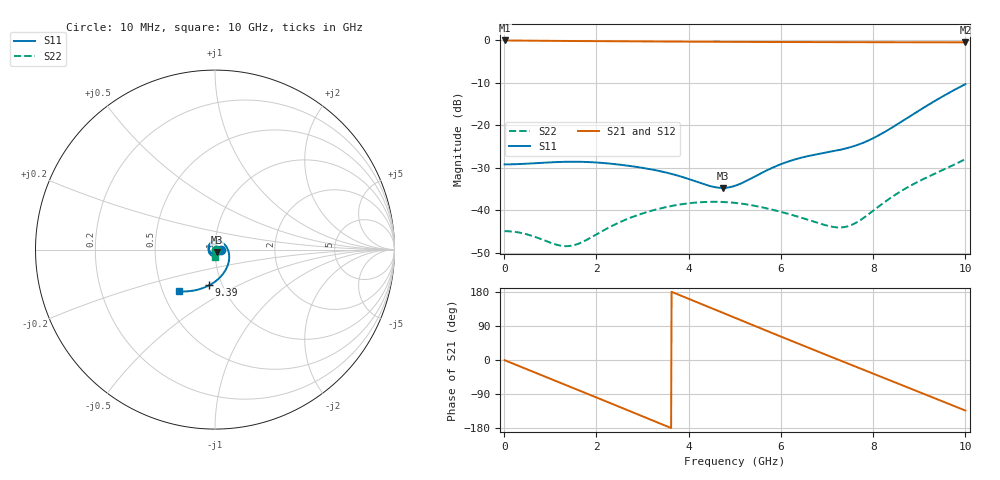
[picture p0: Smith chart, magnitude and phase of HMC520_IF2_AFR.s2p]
! Analog Devices, Inc.
! 1 Analog Way
! Wilmington, MA 01887
! http://www.analog.com
! Date:  2021-09-07 NN
! Board Name:  EV1HMC520ALC4 Revision A with HMC520ALC4 installed
! File Description:  Automatic Fixture Removal S-Parameters for IF2 Port connector and board loss de-embedding
! File Generation:  Calibrated Network Analyzer
! Chip Part Number:  HMC520A
! Chip Description:  GaAs, MMIC, IQ Mixer
! Chip Frequency:  6 to 10 GHz
! Chip Package:  LCC, 3.9 x 3.9 x 0.9 mm
! IF2 Port:  HMC520ALC4 removed and end of trace left open
!Note:
!  Analog Devices supplies this data as a sample of measured data at the evaluation board
!  ports for this product.  Your particular data for this product may vary.
!  Analog Devices reserves the right to change this data at anytime.
!  All lines below in this file are as is from the Network Analyzer.
!Agilent Technologies,N5245A,MY52451809,A.10.47.06
!Automatic Fixture Removal (AFR)
!Date: Friday, August 27, 2021 5:03:51 AM
!S2P File: Measurements: S11,S21,S12,S22:
# MHz S  RI  R 50
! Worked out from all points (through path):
!   1000 points, 10 MHz to 10 GHz, reference 50 ohm
!   highest |S21| = 0.00 dB at 10 MHz (marker M1); lowest = -0.4 dB at 10 GHz (marker M2)
!   group delay of S21, straight-line fit = 137 ps
!   lowest |S11| = -34.7 dB at 4.74 GHz (marker M3), VSWR 1.04, Z = 51.3 - j1.32 ohm
!   |S11| at or under -10 dB: start of sweep to end of sweep
!   |S22| runs from -48.4 to -27.9 dB; largest |S21 - S12| = 1.4e-15
!   S11 on the Smith chart (normalised r, x): 10 MHz: 1.07, -0.00; 9.39 GHz: 0.87, -0.36; 10 GHz: 0.61, -0.31
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10  0.0348 -0.000509  0.9999 -0.0086  0.9999 -0.0086  0.00571 -8.85e-05
750  0.0172 -0.0318  0.7924 -0.5968  0.7924 -0.5968  0.00153 -0.00446
1230  -0.00554 -0.0368  0.4833 -0.8607  0.4833 -0.8607  -0.00252 -0.00292
1680  -0.025 -0.0277  0.1209 -0.9767  0.1209 -0.9767  -0.00409 0.00101
2060  -0.0344 -0.0123  -0.2004 -0.9609  -0.2004 -0.9609  -0.00302 0.00454
2440  -0.0345 0.00557  -0.4991 -0.8421  -0.4991 -0.8421  -0.000141 0.007
2910  -0.0225 0.0232  -0.7897 -0.5724  -0.7897 -0.5724  0.00465 0.00757
3340  -0.00473 0.0289  -0.9413 -0.2429  -0.9413 -0.2429  0.00888 0.00544
4010  0.0178 0.0151  -0.9146 0.3159  -0.9146 0.3159  0.012 -0.00217
4740  0.0132 -0.0129  -0.5446 0.7947  -0.5446 0.7947  0.00619 -0.011
5010  0.00324 -0.0193  -0.3438 0.8986  -0.3438 0.8986  0.00191 -0.0121
5400  -0.0145 -0.0198  -0.0253 0.9601  -0.0253 0.9601  -0.00441 -0.0105
5800  -0.0304 -0.00845  0.3017 0.9102  0.3017 0.9102  -0.00862 -0.00556
6210  -0.0364 0.0124  0.5972 0.7486  0.5972 0.7486  -0.00895 0.000483
6670  -0.0248 0.037  0.8379 0.461  0.8379 0.461  -0.0058 0.00479
7080  0.00124 0.0491  0.9442 0.1457  0.9442 0.1457  -0.00304 0.00572
7480  0.0342 0.043  0.9379 -0.1775  0.9379 -0.1775  -0.00206 0.00626
7890  0.0648 0.014  0.8206 -0.4861  0.8206 -0.4861  -0.00105 0.00888
8340  0.0792 -0.042  0.5803 -0.7558  0.5803 -0.7558  0.00458 0.0128
8870  0.0516 -0.1255  0.1943 -0.9317  0.1943 -0.9317  0.0182 0.00908
9390  -0.033 -0.1992  -0.2223 -0.9245  -0.2223 -0.9245  0.0253 -0.0117
10000  -0.1988 -0.2332  -0.6514 -0.6912  -0.6514 -0.6912  -0.000995 -0.0402
